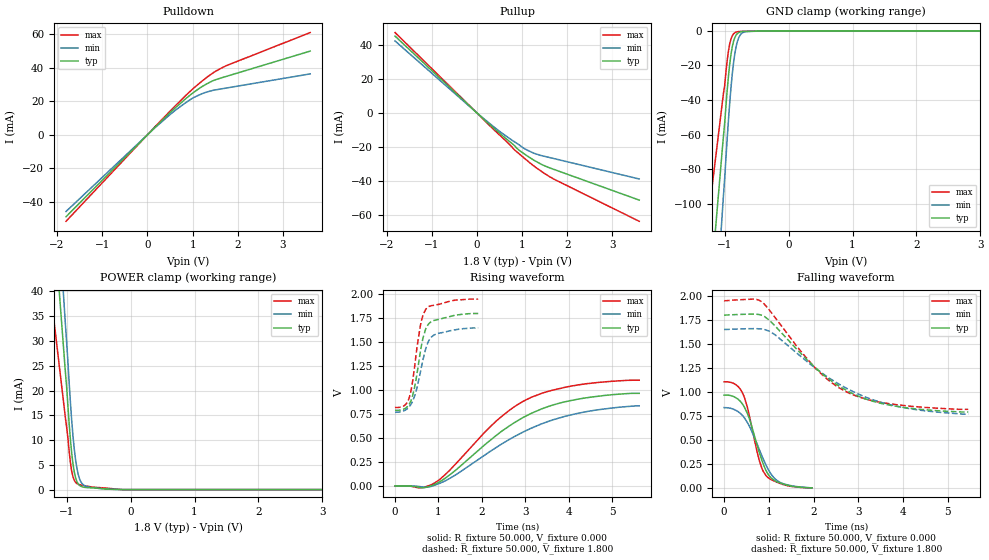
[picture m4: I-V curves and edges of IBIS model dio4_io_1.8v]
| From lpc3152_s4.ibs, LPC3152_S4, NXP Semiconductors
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[Model]   dio4_io_1.8v
Model_type I/O
Vinl=5.400E-01
Vinh=1.260E+00
Vref=0.000E+00
Rref=1.000E+06
Cref=2.500E-11
Vmeas=9.000E-01
C_comp   5.880E-13   5.740E-13   6.020E-13
[Voltage Range]   1.800E+00   1.650E+00   1.950E+00
[POWER Clamp Reference]   1.800E+00   1.650E+00   1.950E+00
[GND Clamp Reference]   0.000E+00   0.000E+00   0.000E+00
[Pullup Reference]   1.800E+00   1.650E+00   1.950E+00
[Pulldown Reference]   0.000E+00   0.000E+00   0.000E+00
[Temperature Range]   25   85   -40
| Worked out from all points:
|   slope of the pulldown table from 0 to 0.27 V, typ, clamps not added: 37.5 ohm
|   slope of the pullup table from 0 to 0.27 V, typ, clamps not added: 41.1 ohm
|   GND clamp passes 1 mA (typ) near -0.78 V on its own axis
|   POWER clamp passes 1 mA (typ) near -0.81 V on its own axis
|   rising waveform, R_fixture 50.000, V_fixture 0.000: 20-80 % time 1.75ns typ, 1.93ns min, 1.57ns max; typ from 0 V to 0.967 V
|   falling waveform, R_fixture 50.000, V_fixture 0.000: 20-80 % time 403ps typ, 483ps min, 342ps max; typ from 0.967 V to 0 V
|   rising waveform, R_fixture 50.000, V_fixture 1.800: 20-80 % time 248ps typ, 284ps min, 220ps max; typ from 0.79 V to 1.8 V
|   falling waveform, R_fixture 50.000, V_fixture 1.800: 20-80 % time 1.51ns typ, 1.72ns min, 1.34ns max; typ from 1.8 V to 0.79 V
[GND Clamp]
-1.8V     -398.7mA   -526.9mA   -273.2mA
-1.02V    -61.16mA   -95.85mA   -36.46mA
-1V       -53.46mA   -85.35mA   -31.62mA
-960mV    -34.18mA   -62.09mA   -16.97mA
-920mV    -18.95mA   -41.24mA   -7.416mA
-880mV    -9.048mA   -24.62mA   -2.803mA
-840mV    -3.793mA   -13mA      -1.088mA
-820mV    -2.405mA   -8.998mA   -753.5uA
-780mV    -1.021mA   -3.989mA   -446.7uA
-740mV    -495.7uA   -1.669mA   -343.6uA
-680mV    -282.4uA   -557.3uA   -249.2uA
3.6V      0A         0A         0A
[Power Clamp]
-1.82V    159.8mA    189.9mA    101.1mA
-1.76V    149.6mA    179.7mA    95.71mA
-1.04V    27.26mA    37.58mA    16.82mA
-980mV    16.97mA    25.89mA    10.45mA
-940mV    10.01mA    17.53mA    5.404mA
-900mV    5.166mA    10.78mA    2.56mA
-880mV    3.553mA    8.176mA    1.877mA
-840mV    1.649mA    4.39mA     1.22mA
-780mV    699.8uA    1.637mA    954.7uA
-680mV    389.1uA    595.5uA    685.6uA
-380mV    108.8uA    93.88uA    309uA
3.6V      0A         0A         0A
[Pullup]
-1.82V    45.38mA    42.52mA    47.49mA
100mV     -2.483mA   -2.267mA   -2.67mA
540mV     -12.84mA   -11.61mA   -13.97mA
840mV     -19.52mA   -17.16mA   -21.95mA
920mV     -21.66mA   -18.53mA   -23.72mA
1.04V     -23.98mA   -20.84mA   -26.44mA
1.3V      -28.43mA   -24.08mA   -32.05mA
1.5V      -31.18mA   -25.58mA   -35.77mA
1.7V      -33.23mA   -26.85mA   -38.95mA
3.6V      -51.4mA    -38.94mA   -63.92mA
[Pulldown]
-1.8V     -48.74mA   -45.64mA   -51.48mA
160mV     4.338mA    4.023mA    4.609mA
600mV     15.66mA    14.24mA    16.84mA
1.02V     25.23mA    22.15mA    27.75mA
1.22V     28.91mA    24.61mA    32.27mA
1.42V     31.84mA    26.28mA    36.29mA
1.74V     34.76mA    27.84mA    41.13mA
3.6V      49.86mA    36.29mA    60.9mA
[Rising Waveform]
R_fixture = 50.000
V_fixture = 0.000
V_fixture_min = 0.000
V_fixture_max = 0.000
|  time   V(typ)   V(min)   V(max)
0s        0V         0V         0V
590ps     -17.68mV   -7.799mV   -19.58mV
940ps     22.85mV    12.02mV    39.76mV
1.43ns    177.6mV    125.4mV    245.8mV
2.335ns   528.8mV    402.8mV    679.1mV
2.76ns    663.9mV    518.1mV    830.5mV
3.135ns   757mV      602.3mV    924.5mV
3.58ns    837mV      681.4mV    994.2mV
4.18ns    903.4mV    755.1mV    1.052V
5.625ns   966.9mV    835.7mV    1.104V
[Falling Waveform]
R_fixture = 50.000
V_fixture = 0.000
V_fixture_min = 0.000
V_fixture_max = 0.000
|  time   V(typ)   V(min)   V(max)
0s        966.9mV    835.7mV    1.104V
250ps     942.3mV    810.7mV    1.079V
430ps     860.5mV    744.1mV    971.1mV
560ps     727.6mV    647.4mV    761.6mV
790ps     365.2mV    396.3mV    282.1mV
855ps     274.8mV    322.8mV    193.6mV
935ps     183mV      239.9mV    129.6mV
1.09ns    89mV       118.9mV    77.49mV
1.245ns   52.03mV    58.89mV    47.01mV
1.965ns   0V         0V         0V
[Rising Waveform]
R_fixture = 50.000
V_fixture = 1.800
V_fixture_min = 1.650
V_fixture_max = 1.950
|  time   V(typ)   V(min)   V(max)
0s        790.2mV    768.2mV    818mV
205ps     802.8mV    784.4mV    835.5mV
330ps     855.1mV    828mV      925.5mV
395ps     925.9mV    875.2mV    1.063V
450ps     1.029V     937.4mV    1.242V
580ps     1.392V     1.179V     1.664V
715ps     1.647V     1.445V     1.848V
820ps     1.71V      1.545V     1.88V
965ps     1.735V     1.589V     1.892V
1.915ns   1.8V       1.65V      1.95V
[Falling Waveform]
R_fixture = 50.000
V_fixture = 1.800
V_fixture_min = 1.650
V_fixture_max = 1.950
|  time   V(typ)   V(min)   V(max)
0s        1.8V       1.65V      1.95V
680ps     1.81V      1.659V     1.966V
840ps     1.798V     1.655V     1.939V
1.15ns    1.682V     1.591V     1.769V
2.06ns    1.244V     1.241V     1.237V
2.355ns   1.13V      1.142V     1.114V
2.79ns    1.002V     1.025V     988mV
3.36ns    897.6mV    912.5mV    904mV
3.865ns   848.9mV    850mV      866.1mV
5.46ns    790.2mV    768.2mV    818mV
[Ramp]
dV/dt_r   5.7779E-01/1.7457E-09   5.0250E-01/1.9234E-09   6.6346E-01/1.5738E-09
dV/dt_f   6.0589E-01/1.5096E-09   5.2908E-01/1.7187E-09   6.7920E-01/1.3430E-09
R_load = 50
